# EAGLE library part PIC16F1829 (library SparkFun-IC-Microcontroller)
PIC16F1829-I/SS SparkFun Products SparkFun Touch Potentiometer (PRT-13144)
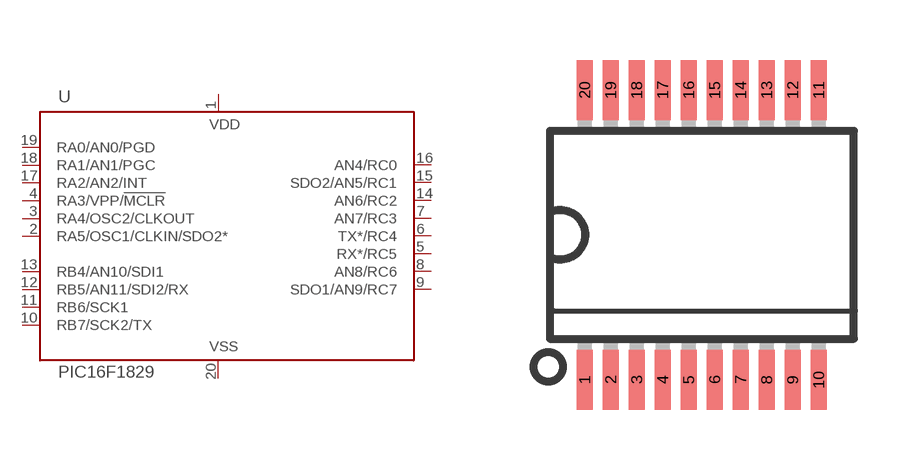
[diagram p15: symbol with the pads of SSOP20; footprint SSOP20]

Designator prefix -

## PIC16F1829 (PROD_ID: IC-12357; VALUE: PIC16F1829-I/SS)  [SSOP20]
1  VDD  pwr
2  RA5/OSC1/CLKIN/SDO2*
3  RA4/OSC2/CLKOUT
4  RA3/VPP/!MCLR  in
5  RX*/RC5
6  TX*/RC4
7  AN7/RC3
8  AN8/RC6
9  SDO1/AN9/RC7
10  RB7/SCK2/TX
11  RB6/SCK1
12  RB5/AN11/SDI2/RX
13  RB4/AN10/SDI1
14  AN6/RC2
15  SDO2/AN5/RC1
16  AN4/RC0
17  RA2/AN2/INT
18  RA1/AN1/PGC
19  RA0/AN0/PGD
20  VSS  pwr

## Footprint SSOP20 (pad centres in mm)
Shrink Small Outline Package package type SS
smd 0.4 x 1.5: 1 -2.925,-3.625; 2 -2.275,-3.625; 3 -1.625,-3.625; 4 -0.975,-3.625; 5 -0.325,-3.625; 6 0.325,-3.625; 7 0.975,-3.625; 8 1.625,-3.625; 9 2.275,-3.625; 10 2.925,-3.625; 11 2.925,3.625; 12 2.275,3.625; 13 1.625,3.625; 14 0.975,3.625; 15 0.325,3.625; 16 -0.325,3.625; 17 -0.975,3.625; 18 -1.625,3.625; 19 -2.275,3.625; 20 -2.925,3.625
